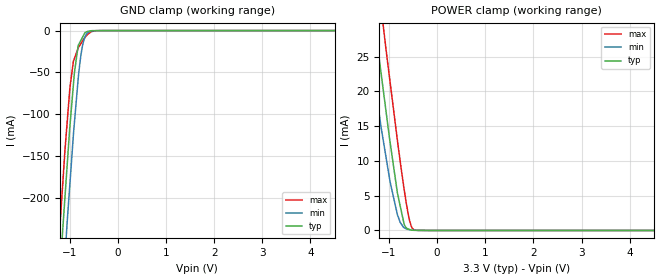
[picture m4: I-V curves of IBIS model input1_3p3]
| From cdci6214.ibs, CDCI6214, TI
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|   input1_3p3 Model
[Model]   input1_3p3
Model_type   Input
Vinl = 0.66
Vinh = 2.64
|   typ   min   max
C_comp   1.095E-12   1.086E-12   1.098E-12
|  Where Nom  PVT is Nominal Process, 3.3V,   32C
|   Fast PVT is Strong Process,  3.465V, -35C
|   Slow PVT is Weak Process,   3.135V,  110C
[Model spec]
|subparameter
Vinl   0.66   0.627   0.693
Vinh   2.64   2.508   2.772
[Voltage Range]   3.3   3.135   3.465
|Junction Temperature
[Temperature Range]   32   110   -35
[Power Clamp Reference]   3.3   3.135   3.465
[GND Clamp Reference]   0   0   0
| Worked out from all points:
|   GND clamp passes 1 mA (typ) near -0.63 V on its own axis
|   POWER clamp passes 1 mA (typ) near -0.69 V on its own axis
[GND Clamp]
|   Voltage   I(typ)   I(min)   I(max)
-3.3V     -2.319A    -2.383A    -2.269A
-1.254V   -335.4mA   -410mA     -276.7mA
-1.147V   -238.5mA   -313.2mA   -183.9mA
-1.099V   -198.7mA   -269.9mA   -142.4mA
-1.057V   -163.2mA   -231.3mA   -111.6mA
-997.3mV  -114.3mA   -183.2mA   -68.51mA
-903.6mV  -50.32mA   -110.2mA   -33.32mA
-824.4mV  -17.71mA   -56.88mA   -20.67mA
-765.7mV  -11.31mA   -28.27mA   -15.22mA
-709.2mV  -5.173mA   -11.71mA   -10.13mA
-627.4mV  -819uA     -2.687mA   -4.556mA
6.6V      0A         0A         0A
[POWER Clamp]
|   Voltage   I(typ)   I(min)   I(max)
-3.3V     150.7mA    135.9mA    169.1mA
-1.593V   46.52mA    36.63mA    57.89mA
-1.391V   35.14mA    25.94mA    45.47mA
-1.331V   31.79mA    23.02mA    41.81mA
-1.247V   27.06mA    18.91mA    36.89mA
-1.161V   22.47mA    14.72mA    31.87mA
-1.047V   16.35mA    9.929mA    25.19mA
-824.4mV  5.363mA    2.264mA    12.92mA
-622.1mV  275.2uA    178.2uA    3.207mA
-538.8mV  50.88uA    76.94uA    637.4uA
-402.1mV  34.3uA     14.68uA    3.844uA
6.6V      0A         0A         0A
